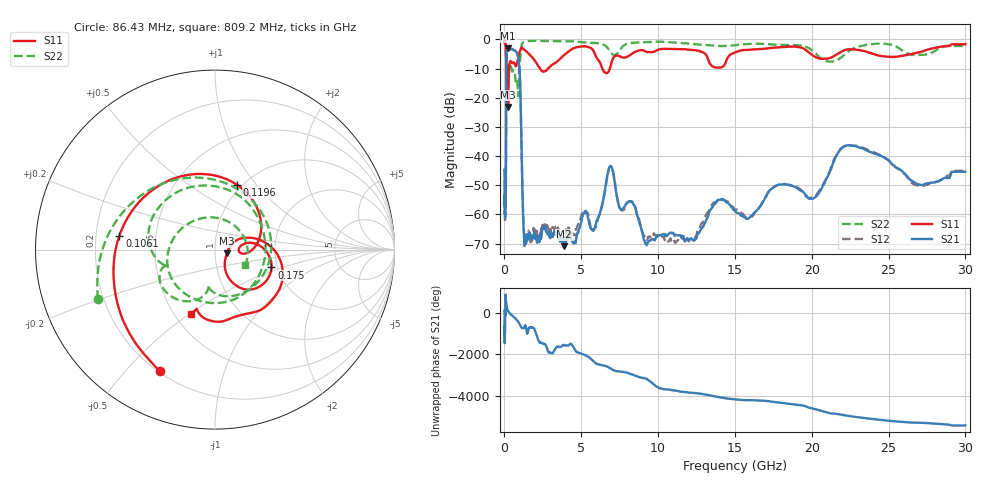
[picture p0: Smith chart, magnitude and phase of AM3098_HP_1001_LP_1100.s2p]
! Date/Time: Thu, Feb 28, 2019 8:41 AM
! Network Analyzer: Agilent Technologies E8364B Rev: A.07.50.67
! Sweep from 0.010 to 30.000 GHz, 1601 Points, Sweep Type: LOG
! Power Supply: 5.023 V, 0.002 A
# Hz S DB R 50
!freq MagS11 AngS11 MagS21 AngS21 MagS12 AngS12 MagS22 AngS22
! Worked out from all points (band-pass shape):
!   1601 points, 10 MHz to 30 GHz, reference 50 ohm
!   highest |S21| = -3.07 dB at 246 MHz (marker M1); lowest = -70.9 dB at 3.875 GHz (marker M2)
!   |S21| within 3 dB of the highest: 130.1 MHz to 886 MHz (756 MHz wide, 149 % of centre)
!   lowest |S11| = -23.2 dB at 239.9 MHz (marker M3), VSWR 1.15, Z = 57 - j2.49 ohm
!   |S11| at or under -10 dB: 192.2 MHz to 300.9 MHz (108.7 MHz wide, 44.1 % of centre); 2.325 GHz to 2.837 GHz (512.3 MHz wide, 19.9 % of centre); 6.372 GHz to 6.857 GHz (485.3 MHz wide, 7.34 % of centre)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
!   |S22| runs from -19.5 to -0.5 dB; largest |S21 - S12| = 0.011
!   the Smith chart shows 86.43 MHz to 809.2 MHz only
!   S11 on the Smith chart (normalised r, x): 86.43 MHz: 0.21, -0.63; 106.1 MHz: 0.30, +0.07; 119.6 MHz: 0.95, +0.80; 175 MHz: 1.86, -0.41; 809.2 MHz: 0.60, -0.51
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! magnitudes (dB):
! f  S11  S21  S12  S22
! 10 MHz  -0.4  -44.8  -44.1  -0.6
! 38.04 MHz  -0.5  -60.0  -60.4  -0.9
! 86.43 MHz  -2.6  -57.3  -54.0  -3.0
! 106.1 MHz  -5.4  -28.5  -28.6  -6.9
! 119.6 MHz  -8.4  -11.4  -11.3  -10.2
! 144.7 MHz  -17.2  -4.4  -4.3  -13.3
! 175 MHz  -9.6  -3.7  -3.7  -9.0
! 239.9 MHz  -23.2  -3.1  -3.0  -11.0
! 246 MHz  -22.2  -3.1  -3.0  -10.9
! 550.5 MHz  -8.0  -3.5  -3.5  -10.7
! 809.2 MHz  -8.3  -4.7  -4.7  -14.5
! 1.009 GHz  -4.1  -13.0  -13.0  -7.6
! 1.295 GHz  -3.6  -70.3  -67.1  -0.8
! 2.084 GHz  -8.1  -67.8  -67.1  -0.5
! 3.875 GHz  -5.4  -70.9  -68.0  -0.6
! 5.841 GHz  -4.4  -64.9  -65.2  -1.2
! 6.855 GHz  -10.0  -43.7  -43.6  -3.9
! 7.926 GHz  -6.1  -56.4  -56.3  -1.6
! 12.01 GHz  -3.5  -68.4  -69.2  -1.4
! 20.1 GHz  -5.6  -54.6  -54.1  -4.1
! 22.56 GHz  -3.4  -36.4  -36.3  -3.5
! 30 GHz  -1.7  -45.4  -45.0  -2.3
